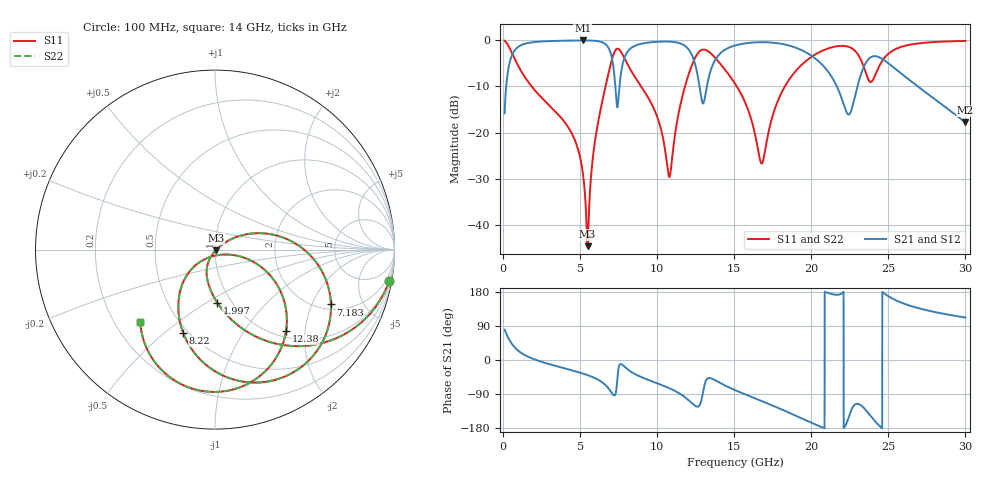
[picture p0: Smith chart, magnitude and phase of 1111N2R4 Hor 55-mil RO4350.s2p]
# GHz S MA R 50
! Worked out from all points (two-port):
!   3201 points, 100 MHz to 30 GHz, reference 50 ohm
!   highest |S21| = -0.05 dB at 5.164 GHz (marker M1); lowest = -17.8 dB at 30 GHz (marker M2)
!   |S21| within 3 dB of the highest: 606.7 MHz to 7.003 GHz (6.396 GHz wide, 168 % of centre); 14.03 GHz to 19.87 GHz (5.836 GHz wide, 34.4 % of centre)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
!   lowest |S11| = -44.6 dB at 5.482 GHz (marker M3), VSWR 1.01, Z = 50.4 - j0.405 ohm
!   |S11| at or under -10 dB: 1.854 GHz to 6.648 GHz (4.794 GHz wide, 113 % of centre); 8.956 GHz to 11.8 GHz (2.848 GHz wide, 27.4 % of centre); 15.17 GHz to 18.29 GHz (3.12 GHz wide, 18.7 % of centre)
!   |S22| runs from -44.6 to -0.1 dB; largest |S21 - S12| = 0
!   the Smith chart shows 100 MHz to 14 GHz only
!   S11 on the Smith chart (normalised r, x): 100 MHz: 1, -11; 1.997 GHz: 0.86, -0.56; 7.183 GHz: 2.24, -2.80; 8.22 GHz: 0.47, -0.58; 12.38 GHz: 1.11, -1.59; 14 GHz: 0.31, -0.37
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0.1  0.9868 -10.1  0.1618 79.9  0.1618 79.9  0.9868 -10.1
0.6325937  0.6947 -50.7  0.7186 39.3  0.7186 39.3  0.6947 -50.7
1.996781  0.2957 -87.5  0.9538 2.3  0.9538 2.3  0.2957 -87.5
5.089563  0.04519 -119.5  0.9944 -34.7  0.9944 -34.7  0.04519 -119.5
5.164313  0.03767 -119.1  0.9944 -35.6  0.9944 -35.6  0.03767 -119.1
5.482  0.005901 -42.8  0.9935 -40.0  0.9935 -40.0  0.005901 -42.8
6.033281  0.09597 33.4  0.9825 -49.3  0.9825 -49.3  0.09597 33.4
7.182563  0.7149 -25.3  0.4776 -93.0  0.4776 -93.0  0.7149 -25.3
7.575  0.7807 -71.5  0.344 -11.7  0.344 -11.7  0.7807 -71.5
8.219719  0.4971 -110.9  0.8003 -28.9  0.8003 -28.9  0.4971 -110.9
10.06978  0.1374 -141.2  0.9633 -62.3  0.9633 -62.3  0.1374 -141.2
10.81728  0.03362 -69.1  0.9654 -74.9  0.9654 -74.9  0.03362 -69.1
12.37769  0.6026 -48.9  0.6119 -118.3  0.6119 -118.3  0.6026 -48.9
12.98503  0.7927 -88.7  0.2069 -82.4  0.2069 -82.4  0.7927 -88.7
14.0035  0.5793 -135.9  0.6951 -58.8  0.6951 -58.8  0.5793 -135.9
15.05  0.3393 -158.6  0.8774 -79.5  0.8774 -79.5  0.3393 -158.6
16.78794  0.04627 -105.7  0.9521 -108.4  0.9521 -108.4  0.04627 -105.7
20.03956  0.6655 -82.4  0.6744 -166.1  0.6744 -166.1  0.6655 -82.4
22.41287  0.8494 -132.6  0.157 -153.2  0.157 -153.2  0.8494 -132.6
23.56216  0.4323 -151.3  0.5775 -133.4  0.5775 -133.4  0.4323 -151.3
25.01978  0.7172 -114.2  0.5597 167.8  0.5597 167.8  0.7172 -114.2
30  0.9823 -160.8  0.129 112.1  0.129 112.1  0.9823 -160.8
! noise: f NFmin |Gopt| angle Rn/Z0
0.1  0.001657  0.8977  3.078  0.003535
3.417  0.01082  0.5204  27.51  0.003748
6.743  0.08528  0.8583  48.34  0.1073
10.06  0.06728  0.757  70.35  0.03777
13.39  0.399  0.942  89.89  0.7726
16.7  0.1116  0.7705  107.8  0.03549
20.03  0.1797  0.8287  123.5  0.05095
23.35  0.572  0.9341  140.1  0.2274
26.67  0.2978  0.8673  153  0.02867
30  0.4475  0.9109  166  0.01878
